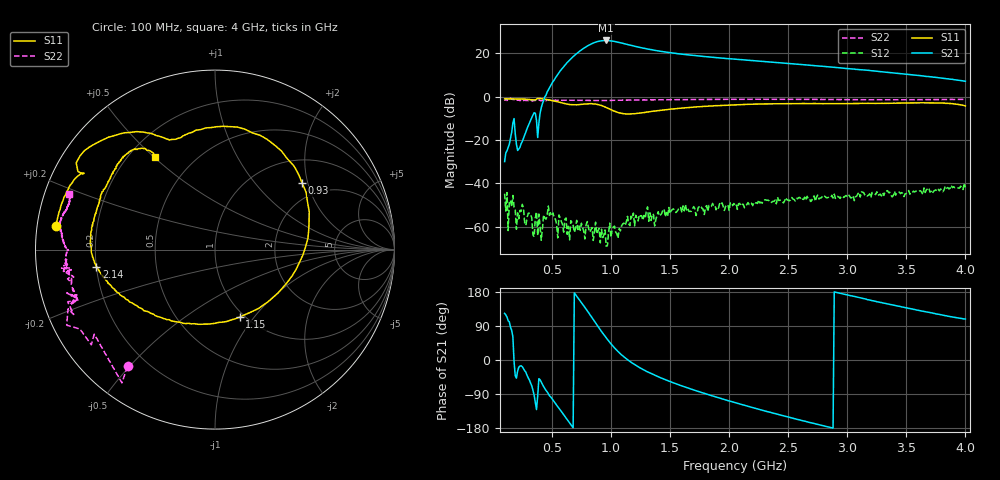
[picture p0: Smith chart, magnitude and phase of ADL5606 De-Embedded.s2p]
! Created Thu Jul 21 11:19:15 2011
# hz S db R 50
! 2 Port Network Data from SP1.SP block
! freq  dbS11  angS11  dbS21  angS21  dbS12  angS12  dbS22  angS22
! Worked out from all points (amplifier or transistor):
!   391 points, 100 MHz to 4 GHz, reference 50 ohm
!   highest |S21| = 26.0 dB at 960 MHz (marker M1)
!   |S21| within 3 dB of that: 787.2 MHz to 1.226 GHz (438.8 MHz wide, 43.6 % of centre)
!   unconditionally stable (mu >= 1): start of sweep to end of sweep
!   at 750 MHz: K = 5.75, MAG = 29.4 dB, |S12| = -58.4 dB
!   at 2.05 GHz: K = 2.39, MAG = 27.0 dB, |S12| = -49.8 dB
!   at 4 GHz: K = 4.48, MAG = 15.0 dB, |S12| = -41.8 dB
!   S11 on the Smith chart (normalised r, x): 100 MHz: 0.06, +0.07; 930 MHz: 1.57, +1.85; 1.15 GHz: 0.95, -0.85; 2.14 GHz: 0.20, -0.07; 4 GHz: 0.31, +0.51
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1e8  -0.96 171.6  -29.91 123.1  -44.69 -111.5  -1.80 -126.8
3.8e8  -0.80 148.0  -18.81 -95.1  -64.04 -126.4  -1.70 -170.2
4.6e8  -1.28 133.4  2.21 -84.1  -54.96 27.4  -1.37 -171.8
6e8  -3.04 116.2  13.93 -144.5  -62.44 61.5  -1.56 -176.2
6.8e8  -3.70 110.0  18.52 -178.8  -59.28 70.2  -1.63 -177.6
7.5e8  -3.53 100.8  21.64 151.4  -58.35 67.9  -1.64 -178.6
7.9e8  -3.34 91.6  23.07 134.0  -58.94 87.6  -1.67 -179.2
8.3e8  -3.17 79.8  24.29 116.3  -61.43 38.2  -1.72 -179.4
8.8e8  -3.48 60.2  25.38 93.4  -63.26 49.1  -1.71 -179.7
9.3e8  -4.28 37.2  25.88 71.1  -64.94 90.7  -1.75 -179.8
9.6e8  -4.94 22.0  25.97 58.7  -68.91 42.7  -1.71 -179.9
1e9  -5.94 1.6  25.77 42.8  -64.90 91.6  -1.68 179.9
1.04e9  -6.88 -19.3  25.41 28.7  -62.43 101.3  -1.62 179.4
1.15e9  -7.94 -69.9  23.97 -1.4  -58.57 98.3  -1.53 178.3
1.25e9  -7.46 -100.7  22.71 -21.4  -55.02 106.0  -1.46 177.3
1.4e9  -6.38 -127.0  21.16 -44.0  -53.01 111.4  -1.39 175.9
1.69e9  -4.84 -152.7  19.11 -78.0  -51.74 93.3  -1.28 173.3
2.05e9  -3.72 -168.6  17.34 -112.4  -49.77 80.6  -1.17 171.0
2.14e9  -3.51 -171.8  16.95 -120.5  -50.46 75.4  -1.15 170.4
2.7e9  -3.12 169.7  14.48 -166.1  -47.77 71.8  -1.22 167.2
3.35e9  -3.03 145.5  11.20 147.6  -44.17 62.8  -1.39 162.6
4e9  -4.24 122.7  7.15 108.1  -41.81 41.2  -1.21 159.2
